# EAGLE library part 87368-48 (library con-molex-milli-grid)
RECEPTACAL
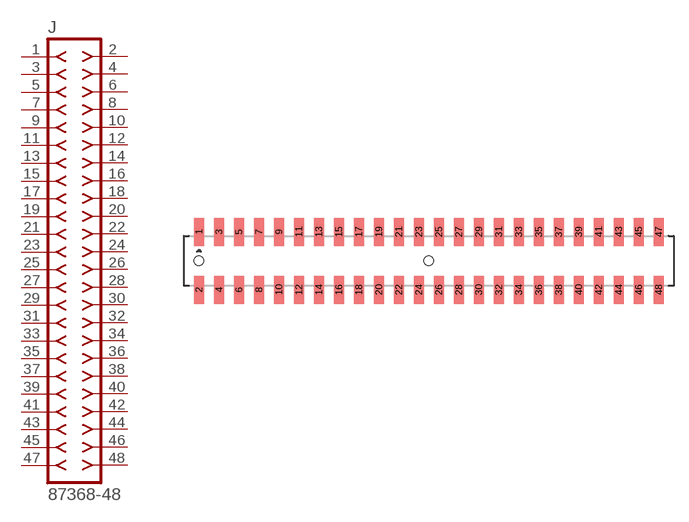
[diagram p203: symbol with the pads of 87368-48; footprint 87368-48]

Designator prefix J

## 87368-48  [87368-48]
1  1  pas
2  2  pas
3  3  pas
4  4  pas
5  5  pas
6  6  pas
7  7  pas
8  8  pas
9  9  pas
10  10  pas
11  11  pas
12  12  pas
13  13  pas
14  14  pas
15  15  pas
16  16  pas
17  17  pas
18  18  pas
19  19  pas
20  20  pas
21  21  pas
22  22  pas
23  23  pas
24  24  pas
25  25  pas
26  26  pas
27  27  pas
28  28  pas
29  29  pas
30  30  pas
31  31  pas
32  32  pas
33  33  pas
34  34  pas
35  35  pas
36  36  pas
37  37  pas
38  38  pas
39  39  pas
40  40  pas
41  41  pas
42  42  pas
43  43  pas
44  44  pas
45  45  pas
46  46  pas
47  47  pas
48  48  pas

## Footprint 87368-48 (pad centres in mm)
RECEPTACAL SMD Dual Row, Side Entry
smd 1 x 2.8: 1 -23,2.9; 2 -23,-2.9; 3 -21,2.9; 4 -21,-2.9; 5 -19,2.9; 6 -19,-2.9; 7 -17,2.9; 8 -17,-2.9; 9 -15,2.9; 10 -15,-2.9; 11 -13,2.9; 12 -13,-2.9; 13 -11,2.9; 14 -11,-2.9; 15 -9,2.9; 16 -9,-2.9; 17 -7,2.9; 18 -7,-2.9; 19 -5,2.9; 20 -5,-2.9; 21 -3,2.9; 22 -3,-2.9; 23 -1,2.9; 24 -1,-2.9; 25 1,2.9; 26 1,-2.9; 27 3,2.9; 28 3,-2.9; 29 5,2.9; 30 5,-2.9; 31 7,2.9; 32 7,-2.9; 33 9,2.9; 34 9,-2.9; 35 11,2.9; 36 11,-2.9; 37 13,2.9; 38 13,-2.9; 39 15,2.9; 40 15,-2.9; 41 17,2.9; 42 17,-2.9; 43 19,2.9; 44 19,-2.9; 45 21,2.9; 46 21,-2.9; 47 23,2.9; 48 23,-2.9
hole 0.914 at -23,0
hole 0.914 at 0,0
